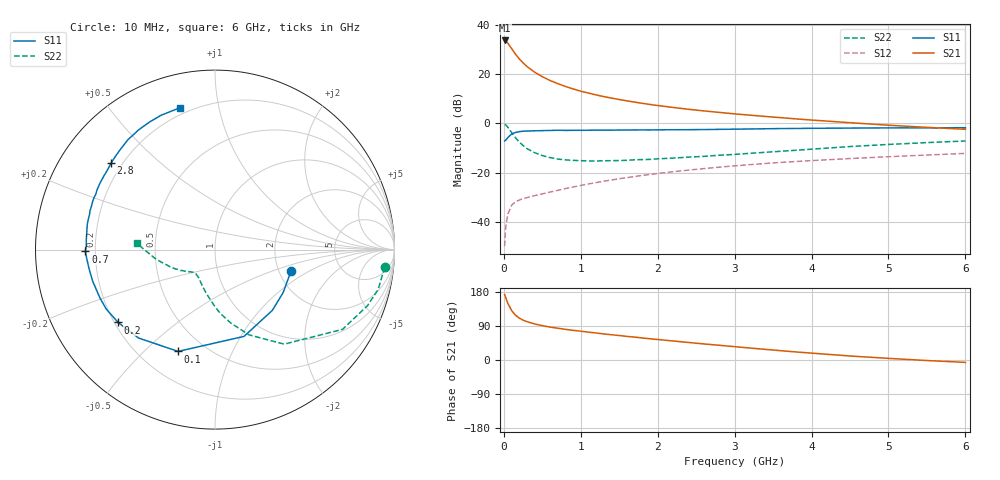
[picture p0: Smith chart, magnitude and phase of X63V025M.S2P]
! SIEMENS Small Signal Semiconductors
! BFP193W
! Si NPN RF Bipolar Junction Transistor in SOT343
! VCE = 3 V  IC = 25 mA
! Common Emitter S-Parameters:  April 1994
# GHz  S  MA  R  50
!  f  S11  S21  S12  S22
! GHz  MAG  ANG  MAG  ANG  MAG  ANG  MAG  ANG
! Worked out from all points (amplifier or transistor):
!   40 points, 10 MHz to 6 GHz, reference 50 ohm
!   highest |S21| = 33.6 dB at 10 MHz (marker M1)
!   |S21| within 3 dB of that: start of sweep to 94.15 MHz
!   unconditionally stable (mu >= 1): 839.4 MHz to 4.061 GHz
!   at 200 MHz: K = 0.41, MSG = 28.7 dB, |S12| = -31.2 dB
!   at 1.5 GHz: K = 1.11, MAG = 14.0 dB, |S12| = -22.5 dB
!   at 6 GHz: K = 0.94, MSG = 4.9 dB, |S12| = -12.2 dB
!   S11 on the Smith chart (normalised r, x): 10 MHz: 2.32, -0.70; 100 MHz: 0.36, -0.64; 200 MHz: 0.21, -0.32; 700 MHz: 0.16, -0.01; 2.8 GHz: 0.16, +0.35; 6 GHz: 0.16, +0.77
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0.01  0.4399 -16.1  48.05 172.7  0.0032 86.7  0.9508 -5.9
0.02  0.4489 -32.2  47.57 167.3  0.0063 79.4  0.9357 -13.7
0.03  0.4655 -46.6  46.33 161.4  0.009 74.1  0.9058 -20.1
0.05  0.5098 -71.5  42.77 150.4  0.014 65.0  0.8384 -32.0
0.1  0.6032 -109.9  33 130.8  0.0216 51.2  0.6528 -53.8
0.15  0.6511 -130.8  25.49 118.4  0.0255 43.9  0.5112 -68.3
0.2  0.6755 -143.1  20.34 110.7  0.0276 41.8  0.4163 -78.1
0.25  0.6907 -151.4  16.86 105.2  0.0295 40.1  0.3545 -85.6
0.3  0.6953 -157.2  14.23 101.2  0.0309 40.3  0.307 -91.4
0.4  0.704 -165.6  10.91 95.1  0.034 41.7  0.2527 -100.4
0.5  0.7095 -171.2  8.838 90.6  0.0369 44.5  0.2211 -107.5
0.6  0.7151 -175.3  7.397 86.9  0.0401 46.7  0.2011 -112.9
0.7  0.7224 -179.2  6.401 83.9  0.0434 48.6  0.1881 -117.1
0.9  0.7194 175.3  4.987 78.3  0.0509 52.0  0.1766 -123.5
1.1  0.7228 170.8  4.108 73.5  0.0587 54.2  0.1718 -128.1
1.6  0.7296 160.5  2.856 62.3  0.0789 56.3  0.1773 -134.9
2.2  0.74 150.1  2.099 50.2  0.1039 55.2  0.1963 -142.0
2.8  0.7532 140.2  1.663 38.8  0.1285 52.5  0.2245 -148.8
3.2  0.7662 134.1  1.461 31.6  0.1446 50.2  0.2457 -154.1
4.5  0.7993 117.0  1.028 10.6  0.1923 41.4  0.3372 -171.5
5.5  0.8082 108.1  0.826 -1.4  0.2267 35.1  0.4052 178.7
6  0.814 104.0  0.755 -6.3  0.2446 32.3  0.4371 175.0
